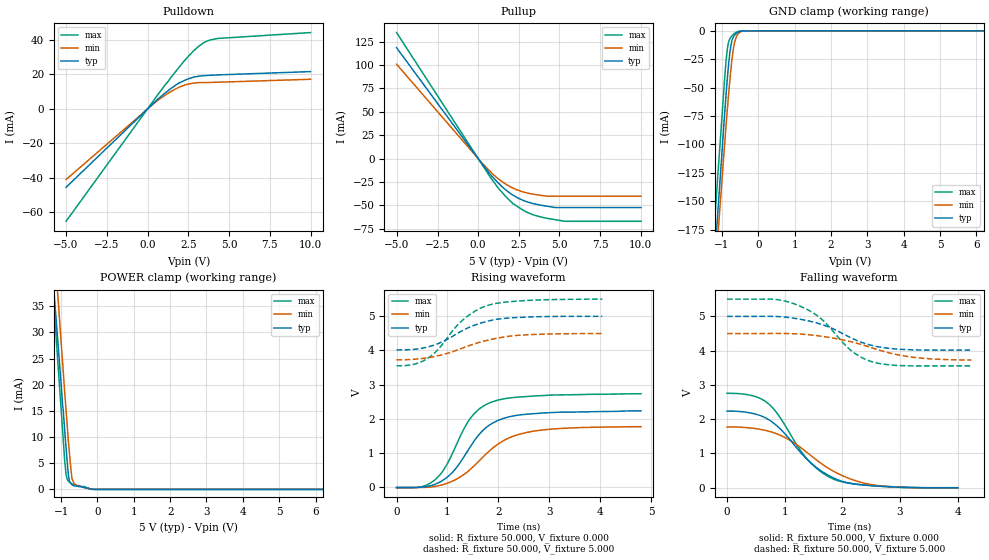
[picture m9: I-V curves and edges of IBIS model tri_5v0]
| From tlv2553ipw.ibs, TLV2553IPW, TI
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[Model]   tri_5v0
Model_type 3-state
Vref=0.000E+00
Rref=5.000E+06
Cref=3.000E-11
Vmeas=2.500E+00
C_comp  2.00000pF 2.00000pF 2.00000pF
[Voltage Range]   5.000E+00   4.500E+00   5.500E+00
[POWER Clamp Reference]   5.000E+00   4.500E+00   5.500E+00
[GND Clamp Reference]   0.000E+00   0.000E+00   0.000E+00
[Pullup Reference]   5.000E+00   4.500E+00   5.500E+00
[Pulldown Reference]   0.000E+00   0.000E+00   0.000E+00
[Temperature Range]   25   105   -40
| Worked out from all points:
|   slope of the pulldown table from 0 to 0.75 V, typ, clamps not added: 113 ohm
|   slope of the pullup table from 0 to 0.75 V, typ, clamps not added: 44 ohm
|   GND clamp passes 1 mA (typ) near -0.55 V on its own axis
|   POWER clamp passes 1 mA (typ) near -0.72 V on its own axis
|   rising waveform, R_fixture 50.000, V_fixture 0.000: 20-80 % time 694ps typ, 871ps min, 613ps max; typ from -0.003 V to 2.24 V
|   falling waveform, R_fixture 50.000, V_fixture 0.000: 20-80 % time 797ps typ, 945ps min, 709ps max; typ from 2.24 V to -0.003 V
|   rising waveform, R_fixture 50.000, V_fixture 5.000: 20-80 % time 824ps typ, 1.01ns min, 743ps max; typ from 4.01 V to 5 V
|   falling waveform, R_fixture 50.000, V_fixture 5.000: 20-80 % time 821ps typ, 1.04ns min, 715ps max; typ from 5 V to 4.01 V
[GND Clamp]
-5V       -1.953A    -1.863A    -1.896A
-1.02V    -114.9mA   -138.8mA   -83.37mA
-900mV    -60.13mA   -87.13mA   -30.11mA
-840mV    -36.37mA   -63.3mA    -12.62mA
-780mV    -17.73mA   -41.54mA   -6.584mA
-740mV    -10.02mA   -28.76mA   -4.697mA
-700mV    -6.018mA   -18.25mA   -3.34mA
-660mV    -3.747mA   -10.62mA   -2.093mA
-560mV    -1.104mA   -2.512mA   -441.3uA
-420mV    -49.77uA   -81.24uA   -7.867uA
0V        83.49uA    136.3uA    13.2uA
10V       83.49uA    136.3uA    13.2uA
[Power Clamp]
-5.02V    382mA      421.1mA    417mA
-1.02V    21.99mA    30.22mA    17.39mA
-960mV    16.26mA    24.36mA    11.42mA
-940mV    14.94mA    22.45mA    9.397mA
-900mV    11.21mA    18.53mA    5.361mA
-860mV    7.716mA    14.82mA    2.616mA
-820mV    4.282mA    11.09mA    1.76mA
-780mV    1.807mA    7.673mA    1.454mA
-700mV    858.5uA    2.062mA    1.002mA
-640mV    636.8uA    1.139mA    853.4uA
-140mV    -7.504uA   -2.687uA   -9.905uA
10.02V    -7.504uA   -2.687uA   -64.33uA
[Pullup]
-5.02V    118.7mA    101mA      134.9mA
200mV     -4.743mA   -4.029mA   -5.306mA
640mV     -14.86mA   -12.03mA   -17.2mA
1.3V      -27.24mA   -22.5mA    -32.96mA
1.62V     -32.47mA   -26.47mA   -39.24mA
2.14V     -39.11mA   -31.64mA   -48.5mA
2.8V      -45.09mA   -35.94mA   -55.62mA
3.38V     -48.3mA    -38.19mA   -60.22mA
4.26V     -51.13mA   -40.36mA   -64.13mA
4.76V     -52.53mA   -40.36mA   -65.55mA
5.34V     -52.53mA   -40.36mA   -67.23mA
10.02V    -52.53mA   -40.36mA   -67.23mA
[Pulldown]
-5V       -45.65mA   -41.12mA   -65.42mA
620mV     5.587mA    4.949mA    8.098mA
1.46V     12.03mA    10.23mA    18.52mA
1.98V     15.33mA    12.78mA    24.74mA
2.82V     18.39mA    14.99mA    33.72mA
3.2V      19.06mA    15.29mA    36.85mA
3.6V      19.39mA    15.29mA    39.24mA
4.32V     19.76mA    15.5mA     40.97mA
10V       21.68mA    17.22mA    44.39mA
[Rising Waveform]
R_fixture = 50.000
V_fixture = 0.000
V_fixture_min = 0.000
V_fixture_max = 0.000
|  time   V(typ)   V(min)   V(max)
0s        -2.571mV   -4.21mV    -14.14mV
480ps     5.661mV    -3.303mV   15.53mV
760ps     92.12mV    28.18mV    227.2mV
1.08ns    410.1mV    170.2mV    934.7mV
1.44ns    1.168V     513.4mV    1.999V
1.64ns    1.578V     802.5mV    2.31V
1.88ns    1.873V     1.139V     2.499V
2.24ns    2.072V     1.464V     2.616V
2.72ns    2.156V     1.649V     2.672V
4.8ns     2.237V     1.773V     2.737V
[Falling Waveform]
R_fixture = 50.000
V_fixture = 0.000
V_fixture_min = 0.000
V_fixture_max = 0.000
|  time   V(typ)   V(min)   V(max)
0s        2.237V     1.773V     2.755V
440ps     2.169V     1.737V     2.685V
720ps     1.988V     1.65V      2.447V
880ps     1.784V     1.56V      2.146V
1.36ns    874.6mV    1.065V     895.5mV
1.6ns     527.7mV    747.9mV    501.2mV
1.84ns    290.4mV    487.2mV    255.5mV
2.12ns    134.2mV    268.6mV    132.1mV
2.56ns    54.55mV    75.82mV    53.73mV
4ns       -2.571mV   -4.21mV    1.547mV
[Rising Waveform]
R_fixture = 50.000
V_fixture = 5.000
V_fixture_min = 4.500
V_fixture_max = 5.500
|  time   V(typ)   V(min)   V(max)
0s        4.015V     3.726V     3.553V
360ps     4.036V     3.745V     3.604V
640ps     4.113V     3.795V     3.799V
840ps     4.216V     3.855V     4.07V
1.12ns    4.432V     3.976V     4.612V
1.28ns    4.571V     4.063V     4.863V
1.52ns    4.733V     4.19V      5.13V
1.76ns    4.845V     4.29V      5.303V
2.48ns    4.971V     4.453V     5.455V
4.04ns    4.998V     4.497V     5.501V
[Falling Waveform]
R_fixture = 50.000
V_fixture = 5.000
V_fixture_min = 4.500
V_fixture_max = 5.500
|  time   V(typ)   V(min)   V(max)
0s        4.998V     4.497V     5.501V
840ps     4.997V     4.5V       5.493V
1.28ns    4.912V     4.481V     5.287V
1.64ns    4.764V     4.418V     4.917V
2.16ns    4.364V     4.255V     3.991V
2.32ns    4.25V      4.184V     3.812V
2.52ns    4.149V     4.078V     3.672V
2.84ns    4.06V      3.923V     3.58V
3.24ns    4.022V     3.804V     3.555V
4.24ns    4.015V     3.726V     3.553V
[Ramp]
| variable typ min max
dV/dt_r 1.34309/707.923p 1.06494/918.989p 1.62954/617.371p
dV/dt_f 589.255m/814.089p 756.903m/1.03230n 1.15596/704.680p
R_load = 50.0000Ohms
